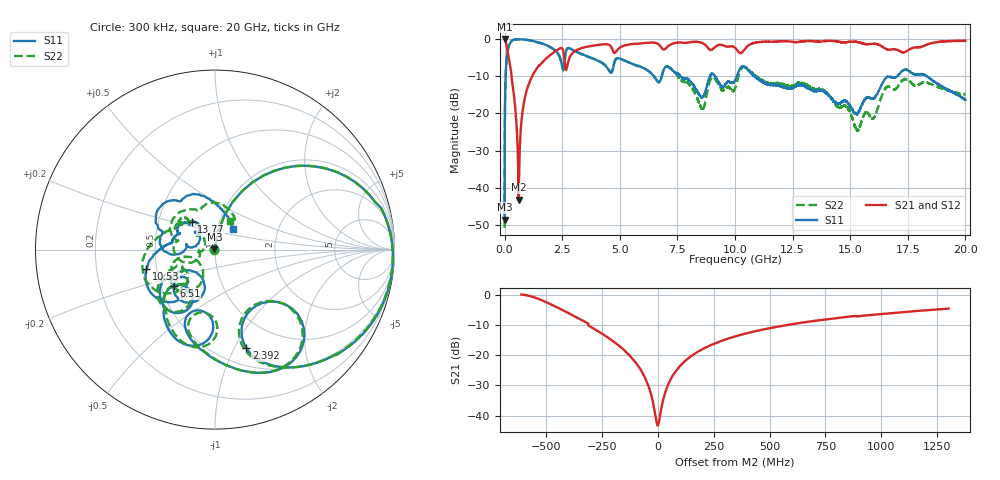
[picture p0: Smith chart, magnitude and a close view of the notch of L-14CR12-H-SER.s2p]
!{L-14CR12}
!Johanson Technology Inc.
!www.johansontechnology.com
!Test Board Conditions:
!Substrate Type  RO4350B
!Substrate Thickness  20 mil
!Substrate Dk  3.66
!TL Type: GCPW
!TL Trace Width  36 mil
!TL Gap  12 mil
!Electrode orientation  Horizontal
!DUT TOPOLOGY	SERIES
!Mounting Pad LxW  26x36 mil
! Created Sun Jun 20 13:10:11 2021
# hz S ma R 50
! 2 Port Network Data from SP1.SP block
! freq  magS11  angS11  magS21  angS21  magS12  angS12  magS22  angS22
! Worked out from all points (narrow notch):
!   20001 points, 300 kHz to 20 GHz, reference 50 ohm
!   highest |S21| = 0.00 dB at 2.3 MHz (marker M1); lowest = -43.3 dB at 611.3 MHz (marker M2)
!   notch at M2: 41.9 dB deep, 217 MHz wide at half that depth
!   lowest |S11| = -48.6 dB at 300 kHz (marker M3), VSWR 1.01, Z = 49.7 + j0.156 ohm
!   |S11| at or under -10 dB: 7.628 GHz to 8.912 GHz (1.284 GHz wide, 15.5 % of centre); 10.85 GHz to 17.05 GHz (6.196 GHz wide, 44.4 % of centre); 18.33 GHz to end of sweep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
!   |S22| runs from -50.8 to -0.1 dB; largest |S21 - S12| = 0.011
!   S11 on the Smith chart (normalised r, x): 300 kHz: 0.99, +0.00; 2.392 GHz: 0.68, -1.12; 6.51 GHz: 0.58, -0.26; 10.53 GHz: 0.44, -0.11; 13.77 GHz: 0.74, +0.24; 20 GHz: 1.18, +0.28
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300000  0.003728 155.0  0.9978 0.1  0.9954 0.0  0.002899 171.2
2300000  0.02025 89.4  0.9997 -1.1  0.9993 -1.2  0.02015 89.1
1.393e8  0.7111 40.8  0.6696 -46.8  0.6715 -46.7  0.7134 40.7
3.213e8  0.9557 13.3  0.2779 -76.2  0.2788 -76.1  0.9585 13.3
6.113e8  0.9937 -5.5  0.00687 -1.6  0.00694 -2.0  0.9925 -5.6
1.0873e9  0.9632 -25.5  0.2666 64.0  0.2665 64.0  0.9593 -25.8
2.3923e9  0.5761 -72.3  0.7497 9.7  0.7494 9.7  0.5703 -73.7
2.6973e9  0.7352 -49.4  0.4068 10.4  0.407 10.3  0.7304 -50.0
3.3343e9  0.6302 -87.1  0.7551 0.7  0.7551 0.7  0.6268 -87.4
6.5103e9  0.3055 -138.6  0.8941 -60.4  0.8951 -60.4  0.3073 -139.9
6.6673e9  0.2645 -129.7  0.8591 -65.7  0.8604 -65.6  0.2639 -131.9
7.1623e9  0.4084 -137.8  0.8307 -60.6  0.8312 -60.5  0.416 -139.8
8.5793e9  0.1659 -124.7  0.8879 -93.3  0.8878 -93.2  0.1146 -143.1
9.0113e9  0.3409 -124.1  0.7226 -91.5  0.7247 -91.6  0.3078 -134.8
1.00003e10  0.2768 -125.3  0.7656 -109.4  0.7653 -109.2  0.2153 -135.2
1.05283e10  0.3968 -164.4  0.7945 -98.0  0.7954 -98.2  0.4003 -173.2
1.33343e10  0.2071 134.6  0.939 -145.7  0.9376 -145.6  0.2191 132.0
1.37733e10  0.2022 130.1  0.9306 -150.8  0.9266 -150.8  0.2115 131.7
1.53103e10  0.09922 160.1  0.9123 -176.2  0.9132 -176.1  0.05845 164.0
1.66673e10  0.31 169.1  0.7177 166.6  0.7125 167.1  0.2308 177.9
1.82273e10  0.3312 110.8  0.8171 164.8  0.82 165.2  0.2624 93.4
2e10  0.1521 49.8  0.9437 134.6  0.9432 134.8  0.1766 62.0
